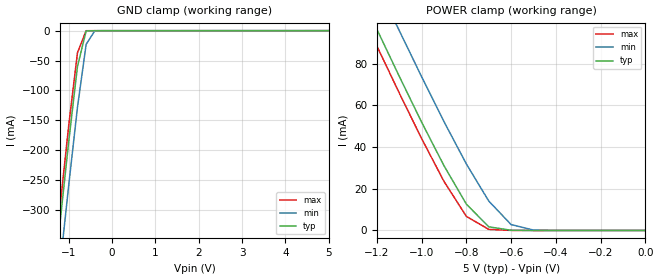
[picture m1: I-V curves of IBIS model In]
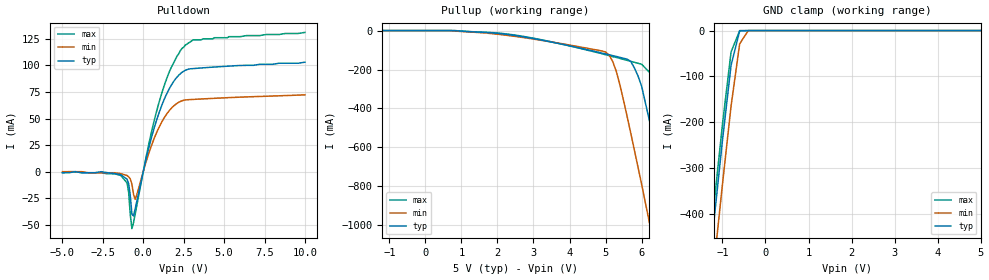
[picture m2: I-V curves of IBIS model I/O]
| IBIS file idt71124.ibs created by s2ibis2 version 1.0
| North Carolina State University Electronics Research Laboratory  1995
[IBIS ver]   2.1
[File name]   idt71124.ibs
[File Rev]   1.0
[Date]   Monday, February 24, 1997
[Source]   HSPICE models at IDT
[Disclaimer]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
[Copyright]   (C) Copyright Integrated Device Technology Corporation 1997
   All rights reserved
|   Component IDT71124S (X step)
[Component]   IDT71124S (X step)
[Manufacturer]   Integrated Device Technology
[Package]
| variable   typ   min   max
R_pkg   100.0m   NA   NA
L_pkg   6.0nH   4.0nH   12.0nH
C_pkg   1.0pF   0.6pF   1.5pF
[Pin]  signal_name   model_name   R_pin   L_pin   C_pin
| in   in   dummy
| ena  enable   dummy
1   A0   In
2   A1   In
3   A2   In
4   A3   In
5   CS#   In
6   I/O0   I/O
7   I/O1   I/O
8   VCC   POWER
9   GND   GND
10   I/O2   I/O
11   I/O3   I/O
12   WE#   In
13   A4   In
14   A5   In
15   A6   In
16   A7   In
17   A8   In
18   A9   In
19   A10   In
20   A11   In
21   A12   In
22   I/O4   I/O
23   I/O5   I/O
24   VCC   POWER
25   GND   GND
26   I/O6   I/O
27   I/O7   I/O
28   OE#   In
29   A13   In
30   A14   In
31   A15   In
32   A16   In
| Models and submodels in the file (2): In (Input), I/O (I/O)
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|   Model In
[Model]   In
Model_type   Input
Vinl =  0.800V
Vinh =  2.200V
C_comp   2.5pF   NA   NA
[Temperature Range]   27.00   100.00   0.000
[Voltage Range]   5.00V   4.50V   5.50V
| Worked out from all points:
|   GND clamp passes 1 mA (typ) near -0.60 V on its own axis
|   POWER clamp passes 1 mA (typ) near -0.65 V on its own axis
[GND_clamp]
| voltage   I(typ)   I(min)   I(max)
-5V       -3.044A    -3.111A    -3.02A
-1.4V     -458mA     -531mA     -432mA
-1.2V     -319mA     -392mA     -293mA
-1V       -184mA     -257mA     -157mA
-800mV    -59.68mA   -128mA     -36.82mA
-600mV    -598uA     -22.84mA   -63.83uA
-400mV    0A         -116uA     0A
5V        0A         191uA      0A
[POWER_clamp]
| voltage   I(typ)   I(min)   I(max)
-5V       1.001A     1.021A     995mA
-1.3V     119mA      141mA      111mA
-1.2V     96.5mA     118mA      88.48mA
-1.1V     73.96mA    95.89mA    65.95mA
-1V       51.94mA    73.73mA    44.08mA
-900mV    31.05mA    52.19mA    23.53mA
-800mV    12.63mA    31.89mA    6.755mA
-700mV    1.754mA    14.11mA    518uA
-600mV    104uA      2.814mA    31.7uA
-500mV    0A         192uA      0A
0V        0A         0A         0A
|   Model I/O
[Model]   I/O
Model_type   I/O
Polarity   Non-Inverting
Enable   Active-High
Vinl =  0.800V
Vinh =  2.200V
C_comp   4.0pF   NA   NA
[Temperature Range]   27.00   100.00   0.000
[Voltage Range]   5.00V   4.50V   5.50V
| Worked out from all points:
|   slope of the pulldown table from 0 to 0.75 V, typ, clamps not added: 16.8 ohm
|   slope of the pullup table from 0 to 0.75 V, typ, clamps not added: 4.98 kohm
|   GND clamp passes 1 mA (typ) near -0.60 V on its own axis
[Pulldown]
| voltage   I(typ)   I(min)   I(max)
-5V       -1mA       0A         -1mA
-1.4V     -2.7mA     -1.8mA     -3.4mA
-1V       -7.1mA     -3.6mA     -10.6mA
-900mV    -11.4mA    -4.8mA     -19.8mA
-700mV    -40.23mA   -11.7mA    -53.59mA
-500mV    -34.98mA   -26.01mA   -39.97mA
300mV     19.75mA    15.26mA    22.79mA
900mV     51.89mA    39.21mA    60.97mA
1.6V      77.72mA    57.21mA    93.41mA
2.4V      93.45mA    66.68mA    116mA
3.1V      96.98mA    67.97mA    124mA
10V       103mA      72.27mA    131mA
[Pullup]
| voltage   I(typ)   I(min)   I(max)
-5V       -30.2fA    0A         -31.9fA
1.9V      -12.64mA   -16.68mA   -11.04mA
5V        -120mA     -110mA     -124mA
5.1V      -124mA     -126mA     -129mA
5.3V      -133mA     -211mA     -138mA
5.7V      -159mA     -528mA     -158mA
6V        -286mA     -790mA     -173mA
6.4V      -612mA     -1.153A    -249mA
6.8V      -967mA     -1.526A    -497mA
7.2V      -1.334A    -1.901A    -846mA
7.6V      -1.708A    -2.276A    -1.206A
10V       -3.96A     -4.531A    -3.454A
[GND_clamp]
| voltage   I(typ)   I(min)   I(max)
-5V       -3.957A    -4.059A    -3.92A
-1.4V     -599mA     -695mA     -564mA
-1.2V     -418mA     -514mA     -383mA
-1V       -240mA     -336mA     -205mA
-800mV    -76.03mA   -165mA     -46.77mA
-600mV    -811uA     -28.91mA   -80.94uA
-400mV    0A         -147uA     0A
5V        0A         0A         0A
[POWER_clamp]
| voltage   I(typ)   I(min)   I(max)
-5V       0A         0A         0A
0V        0A         0A         0A
[Ramp]
| variable   typ   min   max
dV/dt_r   1.21/0.39n   1.07/0.48n   1.39/0.35n
dV/dt_f   2.16/0.53n   1.73/0.72n   2.49/0.48n
R_load = 50.00
| End [Model] I/O
| End [Component] IDT71124S (X step)
